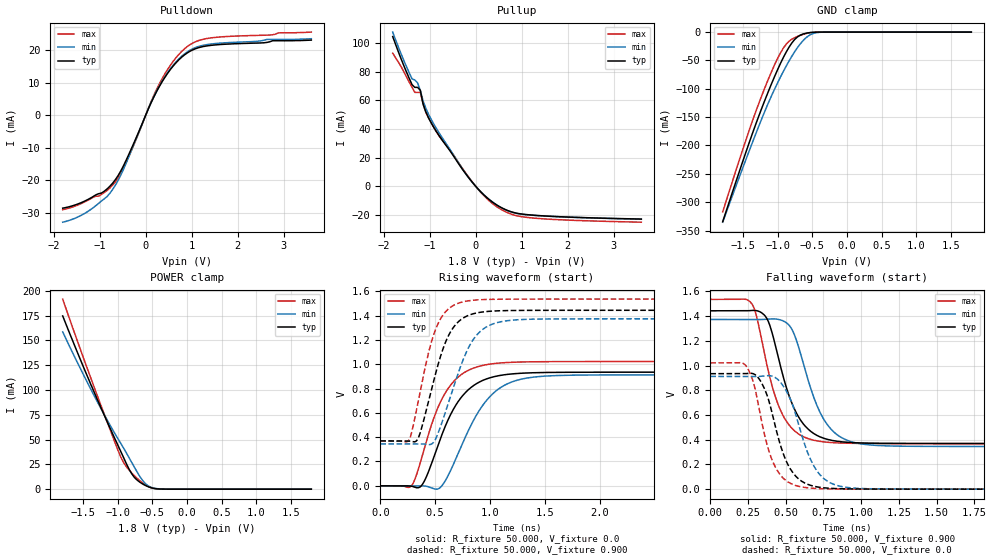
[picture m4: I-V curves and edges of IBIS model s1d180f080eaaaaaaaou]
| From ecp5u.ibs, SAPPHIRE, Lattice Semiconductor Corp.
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|   Model s1d180f080eaaaaaaaou
[Model] s1d180f080eaaaaaaaou
Model_type  Output
Polarity   Non-Inverting
Enable   Active-Low
Vmeas =  0.900V
Cref =  30.000pF
Rref =  50.000
Vref =  0.900V
C_comp   5.000pF   4.000pF   5.500pF
[Temperature Range]   25.000   0.125k   -40.000
[Voltage Range]   1.800V   1.710V   1.890V
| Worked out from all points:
|   slope of the pulldown table from 0 to 0.27 V, typ, clamps not added: 33.1 ohm
|   slope of the pullup table from 0 to 0.27 V, typ, clamps not added: 31.2 ohm
|   GND clamp passes 1 mA (typ) near -0.54 V on its own axis
|   POWER clamp passes 1 mA (typ) near -0.49 V on its own axis
|   rising waveform, R_fixture 50.000, V_fixture 0.0: 20-80 % time 287ps typ, 325ps min, 262ps max; typ from 0 V to 0.934 V
|   rising waveform, R_fixture 50.000, V_fixture 0.900: 20-80 % time 209ps typ, 249ps min, 185ps max; typ from 0.369 V to 1.44 V
|   falling waveform, R_fixture 50.000, V_fixture 0.900: 20-80 % time 167ps typ, 179ps min, 155ps max; typ from 1.44 V to 0.369 V
|   falling waveform, R_fixture 50.000, V_fixture 0.0: 20-80 % time 140ps typ, 159ps min, 125ps max; typ from 0.934 V to 0 V
[Pulldown]
|Voltage   I(typ)   I(min)   I(max)
-1.8V     -28.53mA   -32.84mA   -29.01mA
-1.2V     -25.46mA   -29.03mA   -25.7mA
-900mV    -23.35mA   -25.68mA   -23.75mA
-660mV    -19.84mA   -21.55mA   -20.51mA
-420mV    -13.7mA    -14.59mA   -14.42mA
60mV      2.026mA    2.064mA    2.192mA
240mV     7.384mA    7.52mA     8.023mA
540mV     14.17mA    14.41mA    15.5mA
840mV     18.59mA    18.89mA    20.45mA
1.08V     20.52mA    20.88mA    22.66mA
1.44V     21.61mA    22.02mA    23.91mA
3.6V      23.2mA     23.62mA    25.66mA
[Pullup]
|Voltage   I(typ)   I(min)   I(max)
-1.8V     104.5mA    107.6mA    92.84mA
-1.38V    70.9mA     74.9mA     69.09mA
-1.26V    68.99mA    72.12mA    65.48mA
-1.2V     66.93mA    66.81mA    65.48mA
-1.14V    57.38mA    59.48mA    57.36mA
-1.08V    51.83mA    54.35mA    51.48mA
-900mV    40.67mA    42.94mA    40.69mA
-180mV    7.161mA    7.234mA    7.646mA
360mV     -10.95mA   -10.92mA   -11.94mA
720mV     -17.31mA   -17.4mA    -18.86mA
1.08V     -19.76mA   -19.89mA   -21.68mA
3.6V      -22.97mA   -23.08mA   -25.16mA
[GND_clamp]
|Voltage   I(typ)   I(min)   I(max)
-1.8V     -334.4mA   -335.3mA   -317.1mA
-1.4V     -189.3mA   -204.4mA   -167.3mA
-1.28V    -148.9mA   -166.7mA   -126.7mA
-1.12V    -99.04mA   -119.7mA   -77.45mA
-1V       -64.9mA    -88.2mA    -45.18mA
-920mV    -44.4mA    -68.92mA   -27.88mA
-840mV    -26.71mA   -51.09mA   -16.18mA
-720mV    -8.754mA   -27.82mA   -7.821mA
-640mV    -3.53mA    -15.52mA   -4.188mA
-560mV    -1.27mA    -6.791mA   -1.597mA
-400mV    -49.63uA   -425.4uA   -44.12uA
1.8V      0A         0A         0A
[POWER_clamp]
|Voltage   I(typ)   I(min)   I(max)
-1.8V     174.6mA    158.5mA    191.6mA
-1.36V    100.3mA    96.28mA    105.7mA
-1.12V    62.39mA    65.2mA     61.09mA
-960mV    38.11mA    46.28mA    32.52mA
-880mV    25.96mA    36.75mA    22.79mA
-800mV    15.45mA    26.86mA    16.3mA
-720mV    9.004mA    17.05mA    10.75mA
-640mV    5.132mA    8.487mA    6.134mA
-560mV    2.382mA    3.217mA    2.693mA
-520mV    1.425mA    1.849mA    1.506mA
-360mV    88.16uA    177.6uA    42.1uA
1.8V      0A         0A         0A
[Ramp]
| variable   typ   min   max
dV/dt_r 0.561/0.291n   0.547/0.326n   0.613/0.263n
dV/dt_f 0.564/0.228n   0.550/0.234n   0.620/0.216n
R_load = 50.000
[Rising Waveform]
R_fixture= 50.000
V_fixture= 0.0
V_fixture_min= 0.0
V_fixture_max= 0.0
|time   V(typ)   V(min)   V(max)
0s        0V         0V         0V
292ps     -4.86mV    -190.7uV   9.259mV
392ps     24.06mV    -902.6uV   278.6mV
545ps     382.2mV    -14.42mV   684.7mV
752ps     744.1mV    356.4mV    924.1mV
898ps     851.8mV    616mV      982.6mV
1.038ns   898.1mV    769.1mV    1.006V
1.272ns   925.2mV    874.8mV    1.018V
1.704ns   933.6mV    909.1mV    1.022V
10ns      934.5mV    912.4mV    1.022V
[Rising Waveform]
R_fixture= 50.000
V_fixture= 0.900
V_fixture_min= 0.856
V_fixture_max= 0.946
|time   V(typ)   V(min)   V(max)
0s        369.2mV    344.8mV    368.5mV
265ps     367.6mV    344.8mV    381.3mV
348ps     397.2mV    344.3mV    706.5mV
485ps     859.5mV    357mV      1.241V
564ps     1.109V     528.3mV    1.396V
634ps     1.258V     720.9mV    1.465V
813ps     1.406V     1.154V     1.523V
998ps     1.436V     1.321V     1.533V
1.348ns   1.443V     1.369V     1.536V
10ns      1.443V     1.373V     1.536V
[Falling Waveform]
R_fixture= 50.000
V_fixture= 0.900
V_fixture_min= 0.856
V_fixture_max= 0.946
|time   V(typ)   V(min)   V(max)
0s        1.443V     1.373V     1.536V
281ps     1.447V     1.374V     1.49V
385ps     1.356V     1.377V     952.6mV
450ps     1.07V      1.374V     683.4mV
515ps     781.1mV    1.336V     531mV
617ps     527.2mV    1.016V     424.7mV
767ps     406.1mV    537.3mV    380.8mV
927ps     377.7mV    386.9mV    371.3mV
1.237ns   370.2mV    348.3mV    368.8mV
10ns      369.2mV    344.8mV    368.5mV
[Falling Waveform]
R_fixture= 50.000
V_fixture= 0.0
V_fixture_min= 0.0
V_fixture_max= 0.0
|time   V(typ)   V(min)   V(max)
0s        934.5mV    912.4mV    1.022V
246ps     936.4mV    912.5mV    981.5mV
292ps     930.1mV    911.7mV    836.5mV
351ps     833.7mV    915.7mV    486.3mV
447ps     432.2mV    888.4mV    144.9mV
537ps     151.3mV    709.7mV    43.85mV
667ps     30.08mV    233.8mV    8.455mV
796ps     6.839mV    50.87mV    2.073mV
1.06ns    835.9uV    3.264mV    272.9uV
10ns      0V         0V         0V
